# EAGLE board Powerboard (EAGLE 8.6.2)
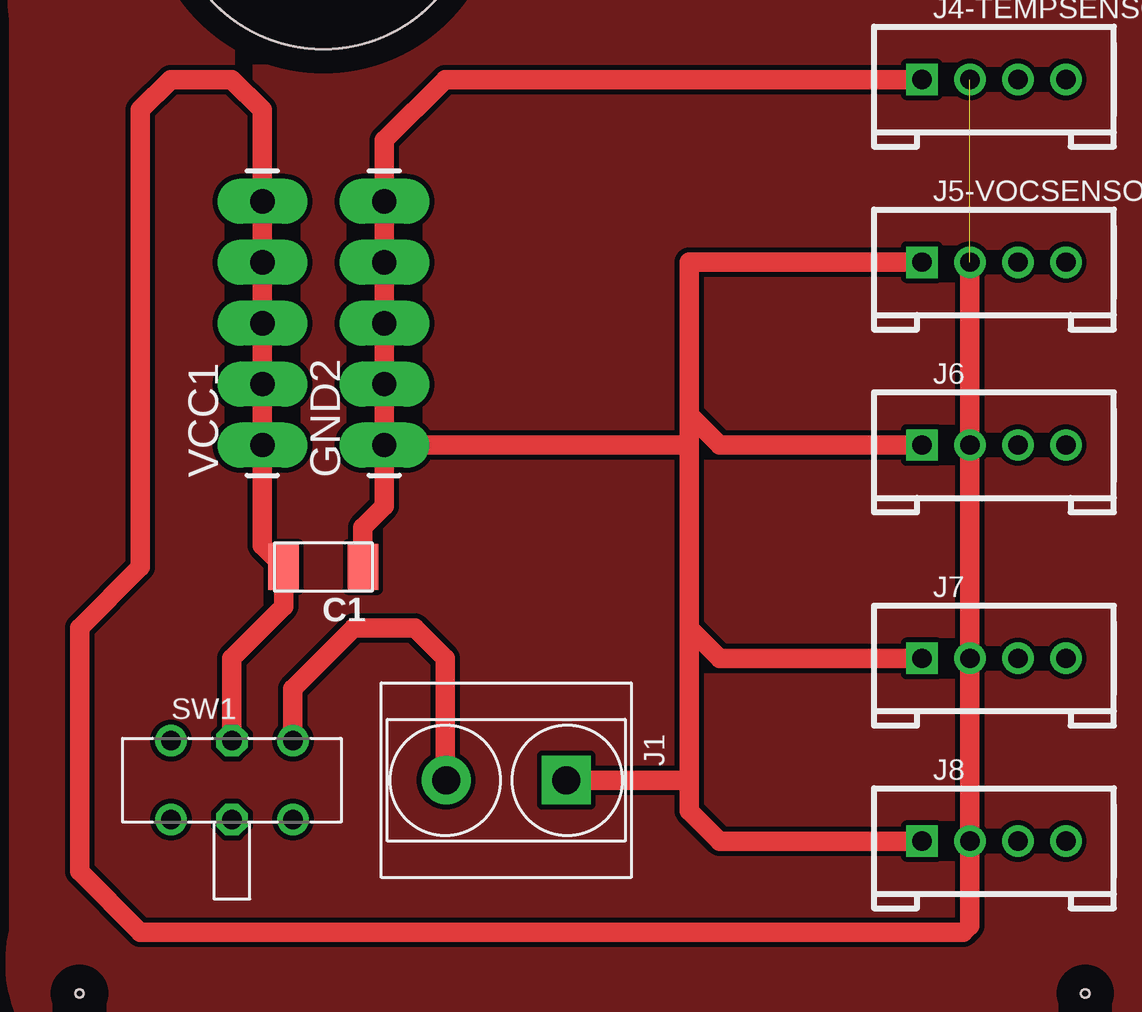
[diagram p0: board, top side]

No outline drawn. Coordinates in mm, seen from the top.
Copper layers (1*16): Top 0.035mm / dielectric 1.5mm / Bottom 0.035mm
Design rules "default": minimum track width 10mil, minimum drill 24mil, track to track 8mil, track to pad 8mil, pad to pad 8mil, via to via 8mil, smd to smd 8mil, copper to edge 40mil, drill to drill 8mil, minimum pad ring 10mil, minimum via ring 8mil, stop-mask expansion 4mil, vias tented up to drill 0mil, thermal gap 10mil
Holes 12.7 mm at 27.94,36.83
Holes 0.35 mm at 59.69,38.1 59.69,-8.89 17.78,-8.89 19.05,36.83

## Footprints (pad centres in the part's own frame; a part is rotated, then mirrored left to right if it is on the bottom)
C1206FAB = smd 1.27 x 1.905: 1 -1.651,0; 2 1.651,0
1X05_LONGPADS = drill 1.016 pad 1.88 long: 1 0,0; 2 2.54,0; 3 5.08,0; 4 7.62,0; 5 10.16,0
H2-5.0-10.5X8.0MM = drill 1.168 pad 2.032 square: 1 0,2.5 | drill 1.168 pad 2.032: 2 0,-2.5
HW4-2.0 = drill 0.8 pad 1.27 square: 1 -3,0 | drill 0.8 pad 1.27: 2 -1,0; 3 1,0; 4 3,0
SW6-2.54-9.0X3.5X3.2MM-90D = drill 0.813 pad 1.27: CH1A -2.54,-1.65; CH1B 2.54,-1.65; CH2A -2.54,1.65; CH2B 2.54,1.65 | drill 0.813 pad 1.27 octagon: COM1 0,-1.65; COM2 0,1.65

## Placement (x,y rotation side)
C1  [C1206FAB]  27.94,8.89 180 top
GND2  [1X05_LONGPADS]  30.48,13.97 90 top
J1  GREEN-2P-5.0  [H2-5.0-10.5X8.0MM]  35.56,0 270 top
J4-TEMPSENSOR  4P-2.0  [HW4-2.0]  55.88,29.21 0 top
J5-VOCSENSOR  4P-2.0  [HW4-2.0]  55.88,21.59 0 top
J6  4P-2.0  [HW4-2.0]  55.88,13.97 0 top
J7  4P-2.0  [HW4-2.0]  55.88,5.08 0 top
J8  4P-2.0  [HW4-2.0]  55.88,-2.54 0 top
SW1  [SW6-2.54-9.0X3.5X3.2MM-90D]  24.13,0 0 top
VCC1  [1X05_LONGPADS]  25.4,13.97 90 top

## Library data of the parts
C1 = fab
GND2 VCC1 = 01_SparkFun
J1 J4-TEMPSENSOR J5-VOCSENSOR J6-J8 = Seeed-Connector
SW1 = Seeed-Switch

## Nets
GND: C1.1 GND2.1 GND2.2 GND2.3 GND2.4 GND2.5 J1.1 J4-TEMPSENSOR.1 J5-VOCSENSOR.1 J6.1 J7.1 J8.1
N$2: J1.2 SW1.CH2B
VCC: C1.2 J4-TEMPSENSOR.2 J5-VOCSENSOR.2 J6.2 J7.2 J8.2 SW1.COM2 VCC1.1 VCC1.2 VCC1.3 VCC1.4 VCC1.5

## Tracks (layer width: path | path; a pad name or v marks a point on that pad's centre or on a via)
GND
  Top 0.813: J5-VOCSENSOR.1 43.18,21.59 43.18,15.24 | J6.1 44.45,13.97 43.18,15.24 | J7.1 44.45,5.08 43.18,6.35 | 43.18,6.35 43.18,13.97 | J8.1 44.45,-2.54 43.18,-1.27 43.18,0 | 43.18,0 43.18,6.35 | 43.18,13.97 43.18,15.24 | GND2.1 43.18,13.97 | GND2.1 GND2.2 GND2.3 GND2.4 GND2.5 | GND2.5 30.48,25.4 | J1.1 43.18,0 | C1.1 29.59,10.54 30.48,11.43 GND2.1 | GND2.5 30.48,26.67 33.02,29.21 J4-TEMPSENSOR.1
N$1
  pour Top: 19.05,-12.7 59.69,-12.7 arc90 64.77,-8.89 64.77,35.28 arc90 58.42,45.5 25.4,45.72 arc90 15.24,31.75 15.24,-6.35 arc90
N$2
  Top 0.813: J1.2 33.02,0.04 33.02,5.08 31.75,6.35 29.21,6.35 26.67,3.81 SW1.CH2B
VCC  (1 unrouted)
  Top 0.813: J5-VOCSENSOR.2 J6.2 J7.2 J8.2 54.88,-6.08 54.61,-6.35 20.32,-6.35 17.78,-3.81 17.78,6.35 20.32,8.89 20.32,27.94 21.59,29.21 24.13,29.21 25.4,27.94 VCC1.5 VCC1.4 VCC1.3 VCC1.2 VCC1.1 25.4,9.78 C1.2 26.29,7.24 24.13,5.08 SW1.COM2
